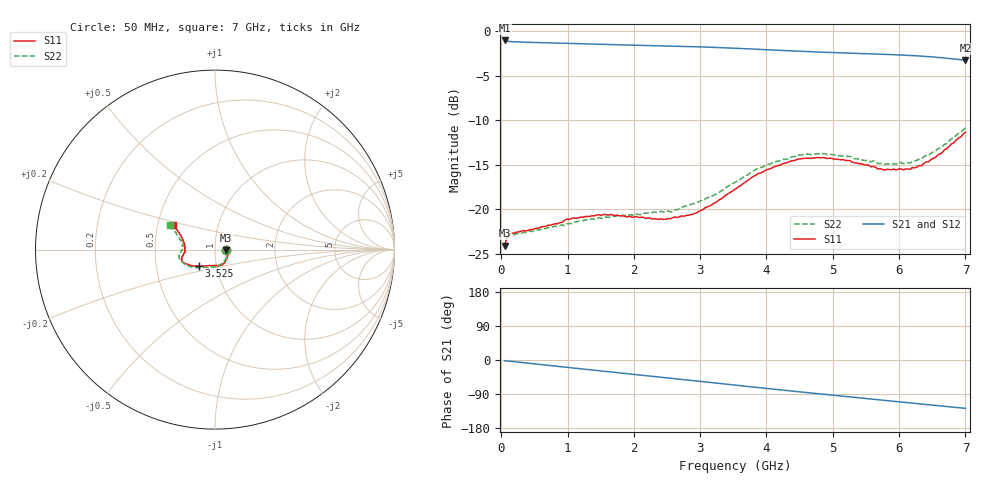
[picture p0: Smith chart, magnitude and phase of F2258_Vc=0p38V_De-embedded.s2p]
! Integrated Device Technology
! Corporate Headquarters
! 6024 Silver Creek Valley Road
! San Jose, CA 95138  USA
! Phone:  1-408-284-8200
! Toll Free:  1-800-223-1366
! Webpage:  http://www.idt.com/
! Timing and RF Division
! 515 Groton Road, Suite 102
! Westford, MA 01886-6024
! Device:  F2258
! Description: Voltage Variable RF Attenuator
! Frequency:  50.0 -  6000.00 MHz
! Package:  3x3 mm Thin QFN Plastic Package: 16 pin
! Ports:  2 RF, 2 DC
!  Pin  1  = NC
!  Pin  2  = NC
!  Pin  3  = RF2  = Port 2
!  Pin  4  = GND
!  Pin  5  = Vdd
!  Pin  6  = NC
!  Pin  7  = VCTRL
!  Pin  8  = NC
!  Pin  9  = GND
!  Pin 10  = RF1  = Port 1
!  Pin 11  = NC
!  Pin 12  = NC
!  Pin 13  = NC
!  Pin 14  = NC
!  Pin 15  = NC
!  Pin 16  = NC
! Vcntrl:  0.380 Volts
! Vdd:  +3.300 Volts
! Current:  1.092 mA
! Data:  The device was measured on a the F2258 evaluation board which has
!  individual transmission lines to the RF pins.  Data was collected
!  using a calibrated network analyzer.  The evaluation board was
!  de-embedded using a TRL calibration technique.
!  The reference plane is the edge of the package pin.
! Misc:  SN 10
!  Action Tracker AT0285
! Date Measured:  2014-12-10
! Date:  2016-01-13  MJV
! Note:
!  Integrated Device Technology supplies this data as a sample of measured
!  data at the package pin for this product.  Your particular data for this
!  product may vary.
!  Data was taken at 25 degrees C.
!  Integrated Device Technology reserves the right to change this data at anytime.
!Freq_(GHz)  S11M_(dB)  S11P_(deg)  S21M_(dB)  S21P_(deg)  S12M_(dB)  S12P_(deg)  S22M_(dB)  S22P_(deg)
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# GHz S dB R 50
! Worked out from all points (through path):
!   201 points, 50 MHz to 7 GHz, reference 50 ohm
!   highest |S21| = -1.01 dB at 50 MHz (marker M1); lowest = -3.2 dB at 7 GHz (marker M2)
!   group delay of S21, straight-line fit = 50.5 ps
!   lowest |S11| = -24.1 dB at 50 MHz (marker M3), VSWR 1.13, Z = 56.7 - j0.415 ohm
!   |S11| at or under -10 dB: start of sweep to end of sweep
!   |S22| runs from -24.1 to -10.8 dB; largest |S21 - S12| = 0.00038
!   S11 on the Smith chart (normalised r, x): 50 MHz: 1.13, -0.01; 3.525 GHz: 0.82, -0.15; 7 GHz: 0.60, +0.18
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0.05  -24.07 -3.3  -1.01 -1.9  -1.01 -1.9  -24.13 -3.0
0.08475  -23.13 -5.6  -1.09 -2.5  -1.09 -2.5  -23.22 -5.2
0.15425  -22.66 -8.6  -1.14 -3.6  -1.15 -3.6  -22.85 -9.1
0.71025  -21.77 -35.0  -1.28 -14.1  -1.28 -14.1  -22.04 -37.3
0.98825  -21.10 -48.4  -1.33 -19.4  -1.33 -19.4  -21.61 -52.9
1.2315  -20.90 -56.4  -1.39 -23.8  -1.39 -23.8  -21.27 -61.9
1.6485  -20.56 -67.9  -1.47 -31.4  -1.47 -31.4  -20.81 -74.9
2.37825  -21.12 -88.6  -1.60 -44.8  -1.60 -44.8  -20.31 -92.9
2.552  -21.06 -94.5  -1.63 -48.0  -1.63 -48.0  -20.29 -98.2
2.93425  -20.43 -111.2  -1.71 -55.1  -1.71 -55.1  -19.35 -111.7
3.247  -19.16 -124.2  -1.79 -61.0  -1.79 -61.0  -18.28 -124.0
3.525  -17.75 -135.0  -1.88 -66.2  -1.88 -66.2  -16.96 -134.6
4.0115  -15.52 -149.2  -2.06 -75.2  -2.06 -75.2  -14.95 -150.2
4.46325  -14.38 -157.9  -2.22 -83.4  -2.22 -83.4  -13.92 -161.4
4.7065  -14.24 -161.2  -2.29 -87.7  -2.29 -87.7  -13.82 -165.7
5.2625  -14.52 -168.1  -2.44 -97.4  -2.44 -97.4  -14.05 -173.8
5.6795  -15.46 -174.7  -2.53 -104.6  -2.53 -104.6  -14.85 -179.3
5.85325  -15.53 -178.9  -2.58 -107.8  -2.58 -107.8  -14.88 176.0
6.166  -15.48 173.3  -2.69 -113.4  -2.69 -113.4  -14.80 170.0
6.33975  -15.08 166.8  -2.77 -116.5  -2.77 -116.5  -14.27 165.6
6.722  -13.17 154.7  -3.00 -123.1  -3.00 -123.1  -12.60 156.6
7  -11.33 149.0  -3.25 -127.4  -3.25 -127.4  -10.83 151.6
